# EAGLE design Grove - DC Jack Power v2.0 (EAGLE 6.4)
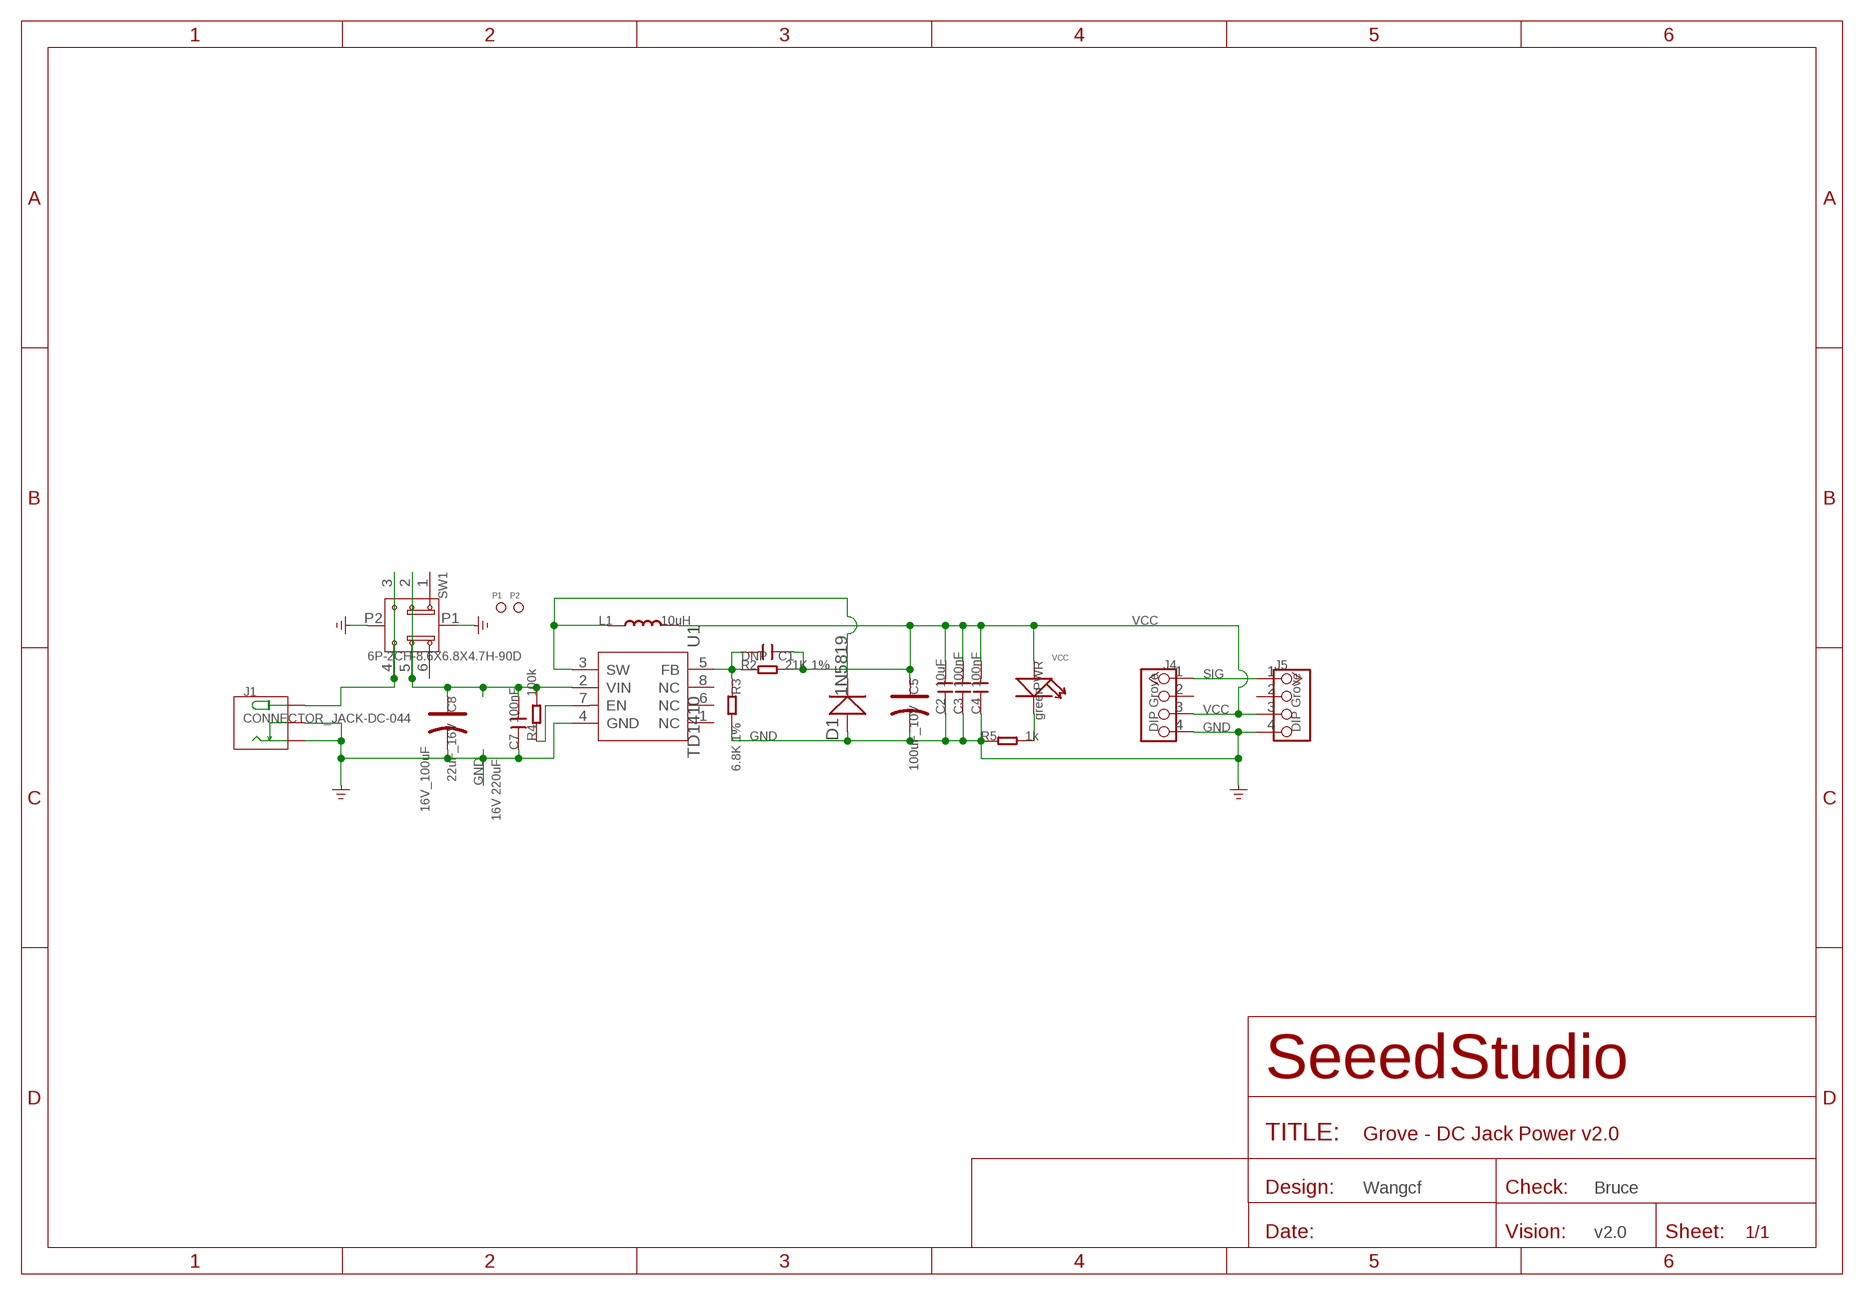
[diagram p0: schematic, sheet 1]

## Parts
C1  DNP  C-0603  [C0603]
C2  10uF  C-0805  [C0805]
C3  100nF  C-0603  [C0603]
C4  100nF  C-0603  [C0603]
C5  100uF_10V  CAP-AVX-B  [AVX-B]
C7  100nF  C-0603  [C0603]
C8  22uF_16V  CAP-AVX-B  [AVX-B]
D1  1N5819  D'SMA'  [DO-214AC]
J1  CONNECTOR_JACK-DC-044  [CONNECTOR_DC-404]
J4  DIP Grove  TWIG-4P-2.0-2.0  [4P-2.0]
J5  DIP Grove  TWIG-4P-2.0-2.0  [4P-2.0]
L1  10uH  L'0630'  [L0630]
P1  PAD-MARK  [ROUND-MARK-1.0]
P2  PAD-MARK  [ROUND-MARK-1.0]
PWR  green  007-LED0603  [D0603]
R2  21K 1%  R-0603  [R0603]
R3  6.8K 1%  R-0603  [R0603]
R4  100k  R-0603  [R0603]
R5  1k  R-0603  [R0603]
SW1  6P-2CH-8.6X6.8X4.7H-90D  SWITCH-2CH-6P-REINFORCE'SK-22D03-G5'  [6P-2CH-8.6X6.8X4.7H-90D]
U1  TD1410  [SOP8]

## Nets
GND: C2.1 C3.1 C4.1 C5.- C7.1 C8.- D1.1(+) J1.- J1.CDN J4.4 J5.4 R3.2 R5.1 SW1.P1 SW1.P2 U1.4(GND)
N$1: PWR.- R5.2
N$2: J1.+ SW1.3 SW1.4
N$52: R4.1 U1.7(EN)
N$53: D1.2(-) L1.1 U1.3(SW)
N$54: C1.2 R2.1 R3.1 U1.5(FB)
SIG: J4.1 J5.1
VCC: C1.1 C2.2 C3.2 C4.2 C5.+ J4.3 J5.3 L1.2 PWR.+ R2.2
VIN: C7.2 C8.+ R4.2 SW1.2 SW1.5 U1.2(VIN)
Unconnected: J4.2 J5.2 SW1.1 SW1.6 U1.1(NC) U1.6(NC) U1.8(NC)

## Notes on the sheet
- 16V_100uF
- 16V 220uF
- Wangcf | Bruce
- v2.0

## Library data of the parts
C1-C4 C7 = Discrete:C*: Ceramic Capacitors
C5 C8 = Discrete:CAP*: Electrolytic Capacitors,Tantalum Capacitors and Super Capacitors
D1 = Discrete:D*
J1 = Grove-DcJackPower:CONNECTOR_JACK-DC-044
J4 J5 = Connector:TWIG-4P-2.0
L1 = Discrete:L*
P1 P2 = Discrete:PAD-MARK; PARTNO: DNP
PWR = Discrete:007-LED*
R2-R5 = Discrete:R*
SW1 = Discrete:SWITCH-2CH-6P-REINFORCE
U1 = template:TD1410: 2A 380KHz 20V PWM Buck DC/DC Converter

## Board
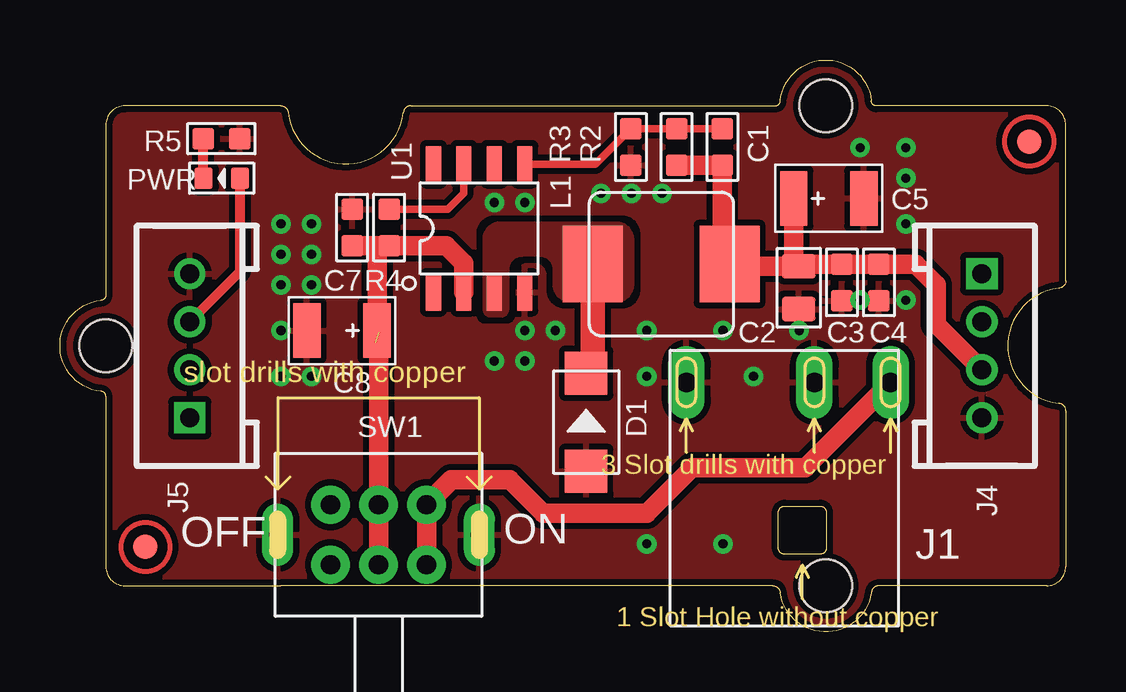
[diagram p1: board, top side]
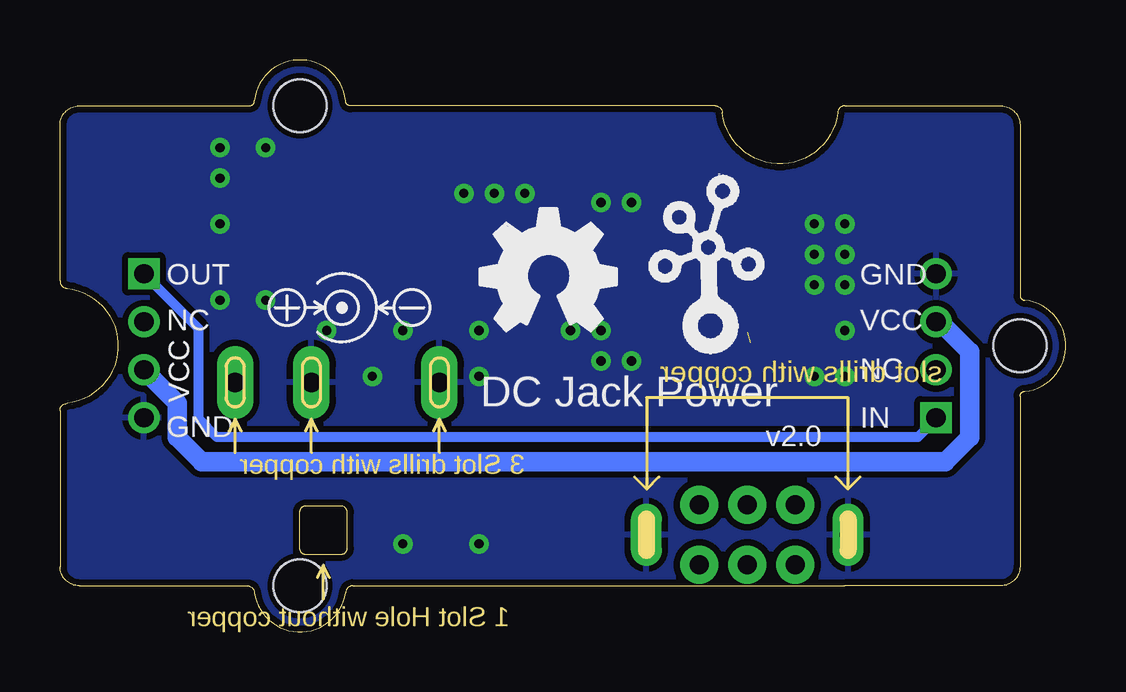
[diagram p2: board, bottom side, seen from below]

Size 41.91 x 23.83 mm. Coordinates in mm from the lower left corner, seen from the top.
Copper layers (1*16): Top 0.035mm / dielectric 1.5mm / Bottom 0.035mm
Design rules "SeeedStudio_2layer_DRU_no_angle_20140221 *": minimum track width 6mil, minimum drill 12mil, track to track 6mil, track to pad 6mil, pad to pad 6mil, via to via 6mil, smd to smd 0mil, copper to edge 10mil, drill to drill 10mil, minimum pad ring 10mil, minimum via ring 6mil, stop-mask expansion 2mil, vias tented up to drill 25mil, thermal gap 10mil

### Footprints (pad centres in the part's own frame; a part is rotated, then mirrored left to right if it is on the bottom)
C0603 = smd 0.889 x 0.889: 1 -0.762,0; 2 0.762,0
C0805 = smd 1.016 x 1.397: 1 -0.889,0; 2 0.889,0
AVX-B = smd 1.143 x 2.286: + -1.46,0; - 1.46,0
DO-214AC = smd 1.8 x 1.77: 1 -2.042,0; 2 2.042,0
CONNECTOR_DC-404 = drill 0.813 pad 1.524 long: + 3.175,10.16; - -5.334,10.16; CDN 0,10.16
4P-2.0 = drill 0.8 pad 1.27 square: 1 -3,0 | drill 0.8 pad 1.27: 2 -1,0; 3 1,0; 4 3,0
L0630 = smd 2.5 x 3.2: 1 -2.85,0; 2 2.85,0
ROUND-MARK-1.0 = smd 1.016 x 1.016: P$1 0,0
D0603 = smd 0.762 x 0.889: + -0.762,0; - 0.762,0
R0603 = smd 0.889 x 0.889: 1 -0.762,0; 2 0.762,0
6P-2CH-8.6X6.8X4.7H-90D = drill 0.8 pad 1.6: 1 -2,1.25; 2 0,1.25; 3 2,1.25; 4 2,-1.25; 5 0,-1.25; 6 -2,-1.25 | drill 0.7 pad 1.3 long: P1 -4.2,0; P2 4.2,0
SOP8 = smd 0.635 x 1.524: 1 -1.905,-2.667; 2 -0.635,-2.667; 3 0.635,-2.667; 4 1.905,-2.667; 5 1.905,2.667; 6 0.635,2.667; 7 -0.635,2.667; 8 -1.905,2.667
GROVE-TEST-PLATFORM = hole 2.2: -10,-10; -10,10; 20,0

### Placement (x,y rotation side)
C1  27.6,20.2 90 top
C2  30.78,14.34 90 top
C3  32.57,14.56 90 top
C4  34.12,14.56 90 top
C5  32.03,18.06 0 top
C7  12.17,16.85 270 top
C8  11.75,12.56 180 top
D1  21.92,8.74 90 top
J1  31.43,0.24 0 top
J4  38.41,11.92 270 top
J5  5.4,11.92 90 top
L1  25.06,15.33 0 top
P1  3.56,3.54 0 top
P2  40.39,20.43 0 top
PWR  6.74,18.91 180 top
R2  25.69,20.2 270 top
R3  23.79,20.2 270 top
R4  13.72,16.84 270 top
R5  6.73,20.56 180 top
SW1  13.27,4.05 0 top
U1  17.46,16.81 0 top
U$3  [OSHW_FILLX200_NOTEXT]  24.39,12.56 0 bottom
U$4  [TWIGLOGO]  14.86,12.56 0 bottom
U$10  [GROVE-TEST-PLATFORM]  21.91,11.92 180 top

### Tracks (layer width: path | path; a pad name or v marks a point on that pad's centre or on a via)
GND  (via drill 0.38 pad 0.81)
  other vias: 33.34,20.18 35.24,20.18 19.37,12.56 24.45,3.67 9.21,12.56 18.1,17.89 19.37,17.89 27.62,12.56 24.45,12.56 35.24,13.83 10.48,10.65 19.37,11.29 10.48,14.46 24.45,10.65 33.34,13.83 30.8,12.56 28.89,10.65 35.24,18.91 35.24,17 20.64,12.56 23.81,18.27 22.54,18.27 25.08,18.27 27.62,3.67 10.48,15.73 9.21,14.46 9.21,10.65 9.21,15.73 18.1,11.29 10.48,17 9.21,17
  pour Bottom (isolate 0.254, rank 2): -0.89,-0.14 44.96,-0.14 44.83,23.99 -1.02,23.99
  pour Top (isolate 0.254, rank 2): -0.89,-0.14 44.96,-0.14 44.83,23.99 -1.02,23.99
N$1
  Top 0.406: PWR.- 5.98,20.55 R5.2
N$2
  Top 0.813: SW1.4 SW1.3 16.31,6.33 18.73,6.33 20.13,4.94 24.45,4.94 26.35,6.84 31.05,6.84 J1.+
N$52
  Top 0.305: R4.1 16.16,17.61 16.83,18.27 U1.7
N$53
  Top 0.203: 22.21,10.93 22.18,10.93 arc45 22.01,10.86 D1.2
  Top 1.016: L1.1 22.21,10.93
  pour Top (isolate 0.254, no thermals): 18.35,13.19 17.97,13.19 arc-90 17.72,13.45 17.72,16.37 arc-90 18.35,17 23.18,17 arc-90 23.81,16.37 23.81,14.46 arc-90 23.18,13.83 21.27,13.83 arc-90 20.64,14.46 20.64,15.1 arc90 20,15.73 19.24,15.73 arc90 18.61,15.1 18.61,13.45 arc-90
N$54
  Top 0.305: R2.1 C1.2 R3.1 22.3,19.48 U1.5
SIG
  Bottom 0.406: J5.1 5.41,8.87 6.16,8.11 35.37,8.11 36.13,8.87 36.13,12.64 J4.1
VCC
  Top 0.406: PWR.+ 7.5,15.02 J5.3
  Top 0.813: J4.3 36.51,12.82 36.51,14.46 35.65,15.32 C4.2 C3.2 30.87,15.32 C2.2 | C5.+ 30.57,15.44 C2.2 | C2.2 27.63,15.23 27.5,15.1 27.68,15.1 L1.2 27.6,15.63 C1.1 R2.2
  Bottom 0.813: J5.3 5.26,12.92 4,11.67 4,8.11 5.02,7.1 36.01,7.1 37.02,8.11 37.02,9.53 J4.3
VIN  (1 unrouted)
  Top 0.813: U1.2 16.83,15.35 16.1,16.08 R4.2 13.15,16.08 | SW1.5 SW1.2 13.27,12.49 C8.+ 13.21,16.02 13.15,16.08 | 13.15,16.08 C7.2 | 13.27,11.92 13.15,12.05

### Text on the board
tPlace: OFF | ON
bPlace: GND | OUT | VCC | NC | NC | VCC | IN | DC Jack Power | v2.0 | GND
